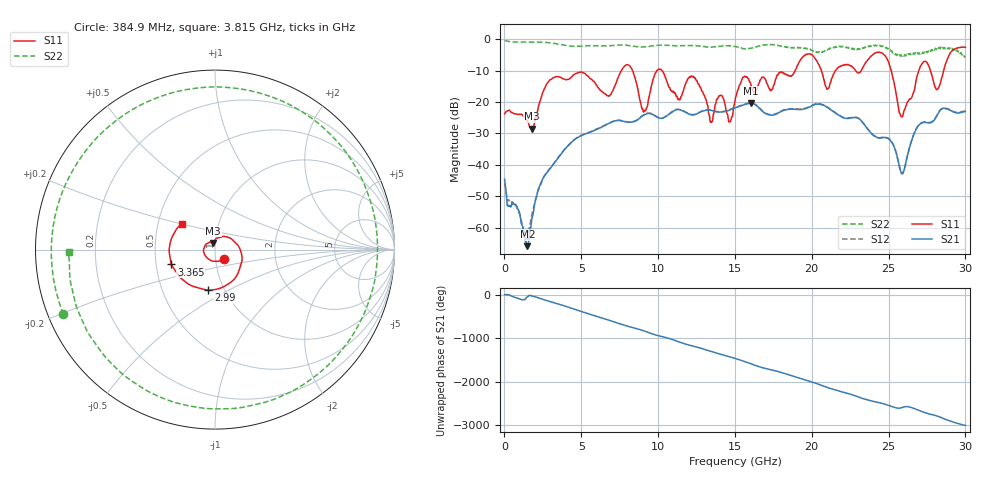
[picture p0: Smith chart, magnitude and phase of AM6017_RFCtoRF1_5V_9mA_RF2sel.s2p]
!Agilent Technologies,E8364B,MY43040894,A.07.50.67
!Agilent E8364B: A.07.50.67
!Date: Tuesday, August 21, 2018 13:34:03
!Correction: S11(Full 2 Port(1,2))
!S21(Full 2 Port(1,2))
!S12(Full 2 Port(1,2))
!S22(Full 2 Port(1,2))
!S2P File: Measurements: S11, S21, S12, S22:
# Hz S  dB  R 50
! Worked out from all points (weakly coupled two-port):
!   1601 points, 10 MHz to 30 GHz, reference 50 ohm
!   highest |S21| = -20.43 dB at 16.04 GHz (marker M1); lowest = -65.9 dB at 1.491 GHz (marker M2)
!   lowest |S11| = -28.5 dB at 1.772 GHz (marker M3), VSWR 1.08, Z = 48.9 + j3.55 ohm
!   |S11| at or under -10 dB: start of sweep to 7.599 GHz; 10.27 GHz to 18.91 GHz (8.642 GHz wide, 59.2 % of centre); 25.17 GHz to 26.96 GHz (1.787 GHz wide, 6.86 % of centre)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
!   |S22| runs from -5.9 to -0.3 dB; largest |S21 - S12| = 0.0024
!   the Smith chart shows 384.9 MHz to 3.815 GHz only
!   S11 on the Smith chart (normalised r, x): 384.9 MHz: 1.10, -0.11; 2.99 GHz: 0.84, -0.40; 3.365 GHz: 0.60, -0.11; 3.815 GHz: 0.66, +0.20
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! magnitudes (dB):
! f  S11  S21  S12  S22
! 10 MHz  -23.7  -44.6  -45.9  -0.3
! 384.9 MHz  -23.0  -53.3  -52.0  -0.7
! 1.491 GHz  -26.0  -65.9  -63.3  -0.8
! 1.772 GHz  -28.5  -57.5  -56.0  -0.8
! 2.99 GHz  -12.8  -41.1  -40.9  -1.1
! 3.365 GHz  -11.8  -38.6  -38.5  -1.4
! 3.815 GHz  -12.6  -35.7  -35.7  -1.8
! 5.015 GHz  -10.4  -30.7  -30.5  -2.2
! 6.795 GHz  -18.1  -26.8  -26.7  -2.0
! 8.089 GHz  -8.2  -26.4  -26.3  -1.9
! 9.082 GHz  -23.0  -24.1  -24.0  -2.4
! 10.02 GHz  -9.5  -25.0  -24.9  -1.9
! 13.43 GHz  -26.4  -22.6  -22.5  -2.5
! 15.01 GHz  -19.5  -21.8  -21.7  -2.3
! 16.04 GHz  -14.4  -20.4  -20.3  -2.9
! 20.01 GHz  -4.9  -21.2  -21.1  -3.4
! 21.02 GHz  -15.9  -21.7  -21.6  -3.4
! 25.01 GHz  -7.5  -31.8  -31.6  -3.1
! 25.84 GHz  -24.6  -42.7  -42.7  -5.1
! 27.02 GHz  -9.2  -27.1  -27.0  -4.5
! 28.18 GHz  -15.9  -24.0  -23.8  -2.7
! 30 GHz  -2.5  -23.0  -22.8  -5.9
